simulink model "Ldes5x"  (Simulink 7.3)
settings: Solver=ode45  StartTime=0.0  StopTime=10.0  RelTol=1e-3
undefined symbols (not defined in the file or in its folder): Als, Bls, Cls, Dls, Kmix

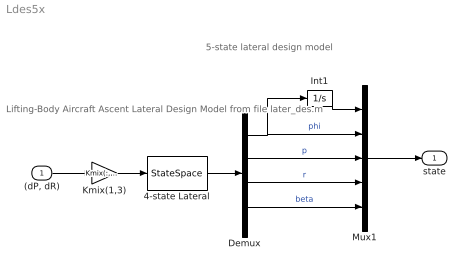
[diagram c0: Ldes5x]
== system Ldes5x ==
  note: 5-state lateral design model
  note: Lifting-Body Aircraft Ascent Lateral Design Model from file later_des.m
  "(dP, dR)" : Inport  OutDataType=sfix(16)  OutScaling=2^0
  4-state Lateral : StateSpace  A=Als  B=Bls  C=Cls  D=Dls
  Demux : Demux
  Int1 : Integrator
  Kmix(1,3) : Gain  Gain=Kmix(:,[1,3])  Multiplication=Matrix(K*u)  ParameterDataType=sfix(16)  ParameterScaling=2^0  OutDataType=sfix(16)  OutScaling=2^0
  Mux1 : Mux  Inputs=5
  state : Outport  OutDataType=sfix(16)  OutScaling=2^0
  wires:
  4-state Lateral/1 -> Demux/1
  "(dP, dR)"/1 -> Kmix(1,3)/1
  Kmix(1,3)/1 -> 4-state Lateral/1
  Demux/2 -> Mux1/3  "p"
  Demux/3 -> Mux1/4  "r"
  Demux/4 -> Mux1/5  "beta"
  Int1/1 -> Mux1/1
  Demux/1 -> Mux1/2, Int1/1  "phi"
  Mux1/1 -> state/1
